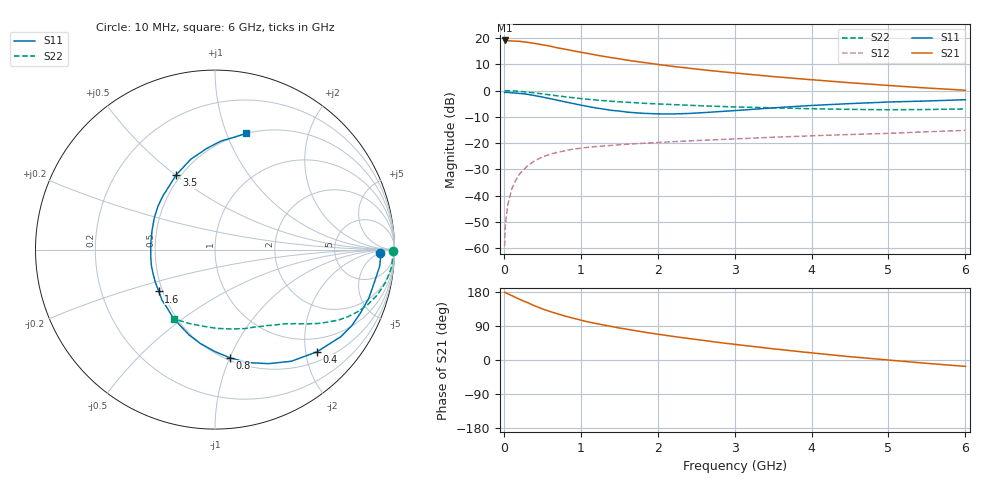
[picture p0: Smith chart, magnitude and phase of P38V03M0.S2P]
! SIEMENS Small Signal Semiconductors
! BFP181
! Si NPN RF Bipolar Junction Transistor in SOT143
! VCE = 8 V  IC = 3 mA
! Common Emitter S-Parameters:  March  1996
# GHz  S  MA  R  50
!  f  S11  S21  S12  S22
! GHz  MAG  ANG  MAG  ANG  MAG  ANG  MAG  ANG
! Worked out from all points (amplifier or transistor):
!   36 points, 10 MHz to 6 GHz, reference 50 ohm
!   highest |S21| = 19.1 dB at 10 MHz (marker M1)
!   |S21| within 3 dB of that: start of sweep to 732.8 MHz
!   unconditionally stable (mu >= 1): 2.244 GHz to end of sweep
!   at 250 MHz: K = 0.16, MSG = 24.4 dB, |S12| = -30.3 dB
!   at 1.4 GHz: K = 0.73, MSG = 16.7 dB, |S12| = -20.8 dB
!   at 6 GHz: K = 1.10, MAG = 5.7 dB, |S12| = -15.1 dB
!   lowest NFmin = 1.40 dB at 450 MHz
!   S11 on the Smith chart (normalised r, x): 10 MHz: 22, -6; 400 MHz: 0.69, -2.23; 800 MHz: 0.52, -1.00; 1.6 GHz: 0.48, -0.26; 3.5 GHz: 0.47, +0.50; 6 GHz: 0.50, +1.17
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0.01  0.9178 -1.3  8.974 178.7  0.0011 89.5  0.9936 -0.4
0.02  0.9238 -2.5  8.93 178.2  0.0028 97.6  0.988 -1.0
0.05  0.9221 -5.8  8.88 175.0  0.0065 91.4  0.9904 -2.8
0.1  0.9056 -12.0  8.793 170.3  0.0131 81.5  0.9888 -5.5
0.2  0.8843 -23.4  8.654 160.7  0.0256 76.3  0.9682 -10.8
0.25  0.8721 -29.0  8.473 156.0  0.0306 72.8  0.9527 -13.3
0.4  0.8042 -45.1  7.888 143.0  0.0462 64.3  0.904 -19.9
0.5  0.7538 -55.6  7.436 134.9  0.0545 58.8  0.8661 -23.6
0.6  0.7023 -64.8  7.015 128.0  0.0617 54.7  0.8282 -26.9
0.7  0.6549 -74.0  6.477 121.7  0.0673 50.6  0.7923 -29.7
0.8  0.6078 -82.3  6.107 115.8  0.072 47.7  0.7601 -31.8
0.9  0.5678 -90.1  5.719 110.4  0.0772 44.8  0.7316 -33.8
1.1  0.4965 -107.0  5.058 100.3  0.0837 40.6  0.6815 -37.2
1.3  0.4435 -122.2  4.462 92.2  0.0884 37.1  0.6427 -40.0
1.6  0.3899 -143.3  3.793 81.3  0.0955 33.8  0.6001 -43.5
1.9  0.3654 -165.8  3.298 71.2  0.1011 31.3  0.566 -47.0
2.2  0.3594 175.2  2.879 62.3  0.1068 29.3  0.5416 -50.7
2.8  0.3985 143.1  2.307 46.2  0.117 26.3  0.5005 -58.7
3.5  0.469 117.4  1.847 29.6  0.1296 22.9  0.4698 -69.5
4.5  0.5651 94.7  1.409 8.7  0.1459 17.9  0.439 -88.8
5.5  0.6345 80.4  1.118 -8.8  0.1646 14.1  0.4366 -109.7
6  0.67 75.0  1.015 -16.9  0.1751 11.4  0.4472 -120.5
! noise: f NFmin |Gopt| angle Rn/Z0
0.45  1.4  0.56  17  0.36
0.9  1.5  0.45  35  0.34
1.8  1.85  0.25  82  0.36
